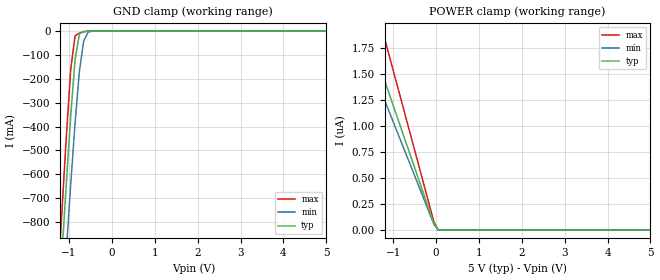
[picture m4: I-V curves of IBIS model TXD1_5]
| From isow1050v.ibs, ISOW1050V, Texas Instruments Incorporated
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|   TXD1_5 Model
[Model]   TXD1_5
Model_type Input
Polarity   Inverting
Enable   Active-High
Vinl =  1.500V
Vinh =  3.500V
C_comp   1.300pF   1.100pF   1.500pF
[Model Spec]
Vinh   3.500V   3.150V   3.850V
Vinl   1.500V   1.350V   1.650V
[Temperature Range]   27.000   0.150k   -55.000
[Voltage Range]   5.000V   4.500V   5.500V
[POWER Clamp Reference]   5.000V   4.500V   5.500V
[GND Clamp Reference]   0.0V   0.0V   0.0V
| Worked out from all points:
|   GND clamp passes 1 mA (typ) near -0.60 V on its own axis
[GND_clamp]
|Voltage   I(typ)   I(min)   I(max)
-5V       -9.985A    -9.609A    -10.4A
-1.263V   -1.229A    -1.49A     -1.058A
-1.162V   -926.6mA   -1.199A    -742.7mA
-1.061V   -632.4mA   -915.1mA   -437.4mA
-960mV    -354.3mA   -640.8mA   -159.9mA
-859mV    -119.3mA   -384.6mA   -19.73mA
-758mV    -11.77mA   -168.2mA   -8.316mA
-657mV    -1.875mA   -40.74mA   -2.94mA
-556mV    -310.1uA   -4.661mA   -414.1uA
-455mV    -23.79uA   -355uA     -18.34uA
5V        0A         0A         -767.5nA
[POWER_clamp]
|Voltage   I(typ)   I(min)   I(max)
-5V       5.989uA    5.198uA    7.677uA
-1.868V   2.237uA    1.943uA    2.868uA
-1.767V   2.116uA    1.838uA    2.713uA
-1.666V   1.995uA    1.733uA    2.558uA
-1.565V   1.875uA    1.628uA    2.403uA
-1.262V   1.512uA    1.313uA    1.938uA
-1.161V   1.391uA    1.208uA    1.782uA
-50mV     59.98nA    53.97nA    76.87nA
51mV      0A         0A         0A
5V        0A         0A         0A
